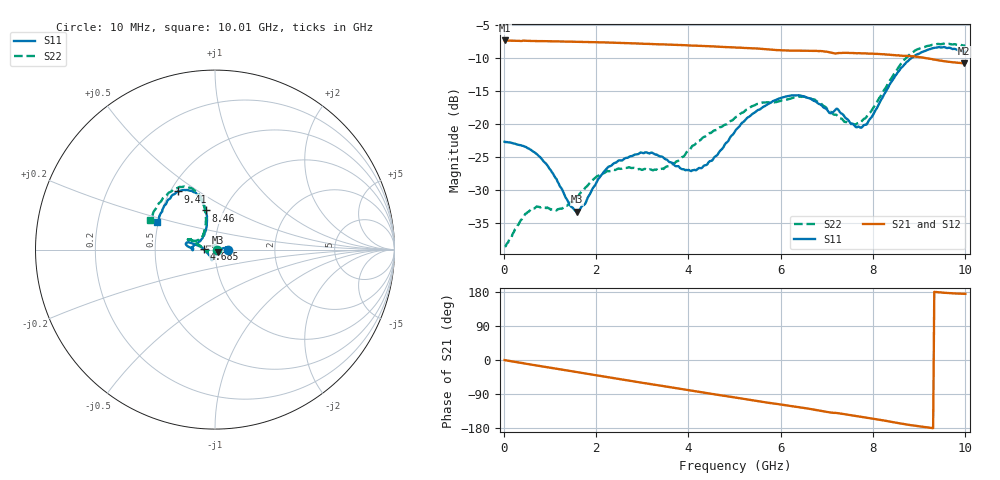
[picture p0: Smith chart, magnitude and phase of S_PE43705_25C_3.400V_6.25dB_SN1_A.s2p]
! Device ID: PE43705
! Serial: 1
! Insertion: A
! Impedance: 50 ohm
! Temp: 25C
! VDD: 3.400V
! Attenuation Step: 6.25dB
#  Hz  S  RI  R  50
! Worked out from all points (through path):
!   401 points, 10 MHz to 10.01 GHz, reference 50 ohm
!   highest |S21| = -7.28 dB at 10 MHz (marker M1); lowest = -10.7 dB at 9.985 GHz (marker M2)
!   group delay of S21, straight-line fit = 53 ps
!   lowest |S11| = -33.3 dB at 1.585 GHz (marker M3), VSWR 1.04, Z = 51.5 - j1.64 ohm
!   |S11| at or under -10 dB: start of sweep to 8.832 GHz
!   |S22| runs from -38.5 to -7.8 dB; largest |S21 - S12| = 0.0039
!   S11 on the Smith chart (normalised r, x): 10 MHz: 1.16, -0.00; 4.685 GHz: 0.88, +0.00; 8.46 GHz: 0.83, +0.38; 9.41 GHz: 0.55, +0.42; 10.01 GHz: 0.49, +0.18
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1e7  0.0735 -0.000231  0.4326 -0.00206  0.4329 -0.00203  0.0118 0.000267
4.6e8  0.0665 0.0112  0.4239 -0.0712  0.424 -0.0704  0.00923 0.0187
7.6e8  0.0556 0.0123  0.412 -0.1146  0.4121 -0.1143  0.00147 0.0235
1.185e9  0.0353 0.00178  0.3883 -0.1731  0.3882 -0.1729  -0.013 0.0186
1.585e9  0.0146 -0.0159  0.3579 -0.2242  0.3581 -0.224  -0.0271 0.00661
1.685e9  0.0103 -0.0216  0.3495 -0.2361  0.3496 -0.2359  -0.0307 0.00308
2.31e9  -0.00763 -0.0475  0.287 -0.3022  0.287 -0.302  -0.0421 -0.0131
2.96e9  -0.017 -0.0585  0.2083 -0.3523  0.2086 -0.352  -0.0436 -0.0126
3.36e9  -0.0183 -0.0544  0.1575 -0.3727  0.158 -0.3722  -0.0437 -0.0106
4.11e9  -0.0368 -0.0255  0.0576 -0.3916  0.0581 -0.3915  -0.0686 0.00817
4.685e9  -0.0627 0.00242  -0.0192 -0.3864  -0.0184 -0.3865  -0.0916 0.0254
5.01e9  -0.0861 0.0195  -0.0597 -0.3778  -0.0593 -0.3782  -0.1062 0.0351
5.96e9  -0.1508 0.0412  -0.1636 -0.3266  -0.1624 -0.3266  -0.1383 0.0557
6.685e9  -0.1521 0.0182  -0.2323 -0.2756  -0.2322 -0.2757  -0.1449 0.0551
7.435e9  -0.1053 0.0319  -0.2815 -0.205  -0.2808 -0.2058  -0.0859 0.0585
7.735e9  -0.073 0.059  -0.2987 -0.1745  -0.2975 -0.1752  -0.0663 0.0785
8.36e9  -0.0459 0.1928  -0.3212 -0.1029  -0.3204 -0.1039  -0.0536 0.2056
8.46e9  -0.0504 0.2179  -0.3221 -0.0895  -0.3216 -0.0911  -0.0579 0.2335
8.885e9  -0.1015 0.308  -0.3253 -0.0408  -0.3232 -0.0423  -0.1193 0.3344
9.41e9  -0.2058 0.3237  -0.3066 0.00596  -0.3062 0.00558  -0.228 0.338
9.985e9  -0.3133 0.164  -0.2892 0.0274  -0.2897 0.0273  -0.3531 0.176
1.001e10  -0.3205 0.1548  -0.2903 0.0276  -0.2914 0.0275  -0.3609 0.1648
